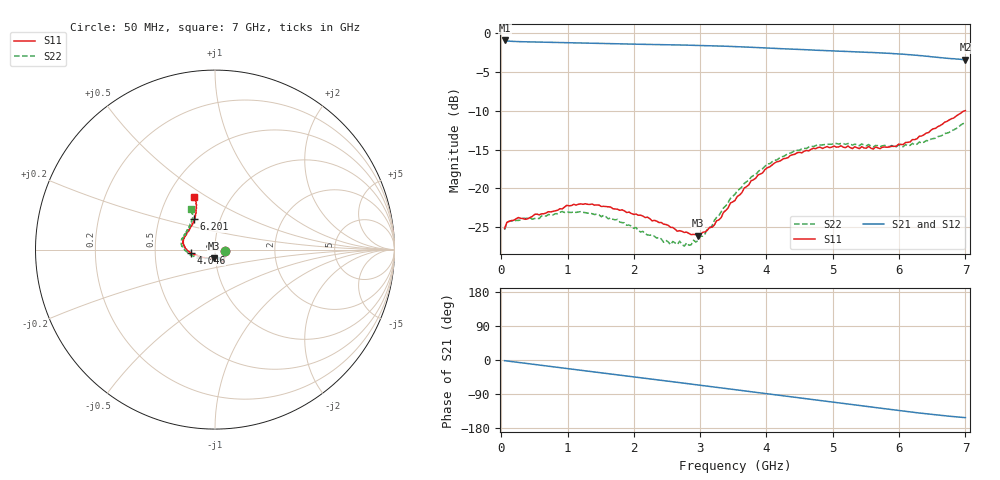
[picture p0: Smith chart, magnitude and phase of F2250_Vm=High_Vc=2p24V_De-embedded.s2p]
! Integrated Device Technology
! Corporate Headquarters
! 6024 Silver Creek Valley Road
! San Jose, CA 95138  USA
! Phone:  1-408-284-8200
! Toll Free:  1-800-223-1366
! Webpage:  http://www.idt.com/
! Timing and RF Division
! 515 Groton Road, Suite 102
! Westford, MA 01886-6024
! Device:  F2250
! Description: Voltage Variable RF Attenuator
! Frequency:  50.0 -  6000.00 MHz
! Package:  3x3 mm Thin QFN Plastic Package: 16 pin
! Ports:  2 RF, 3 DC
!  Pin  1  = GND
!  Pin  2  = NC
!  Pin  3  = RF1  = Port 1
!  Pin  4  = NC
!  Pin  5  = GND
!  Pin  6  = GND
!  Pin  7  = GND
!  Pin  8  = GND
!  Pin  9  = NC
!  Pin 10  = RF2  = Port 2
!  Pin 11  = NC
!  Pin 12  = GND
!  Pin 13  = GND
!  Pin 14  = VCNTRL
!  Pin 15  = VDD
!  Pin 16  = VMODE
! Vcntrl:  2.240 Volts
! Vmode:  +3.300 Volts
! Vdd:  +3.30  Volts
! Current:  1.315 mA
! Data:  The device was measured on a the F2250 evaluation board which has
!  individual transmission lines to the RF pins.  Data was collected
!  using a calibrated network analyzer.  The evaluation board was
!  de-embedded using a TRL calibration technique.
!  The reference plane is the edge of the package pin.
! Misc:  SN 10
!  Action Tracker AT0258
! Date Measured:  2014-11-26
! Date:  2015-10-15  MJV
! Note:
!  Integrated Device Technology supplies this data as a sample of measured
!  data at the package pin for this product.  Your particular data for this
!  product may vary.
!  Data was taken at 25 degrees C.
!  Integrated Device Technology reserves the right to change this data at anytime.
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# GHz S dB R 50
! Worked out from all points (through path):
!   201 points, 50 MHz to 7 GHz, reference 50 ohm
!   highest |S21| = -0.92 dB at 50 MHz (marker M1); lowest = -3.4 dB at 7 GHz (marker M2)
!   group delay of S21, straight-line fit = 61.1 ps
!   lowest |S11| = -26.1 dB at 2.969 GHz (marker M3), VSWR 1.10, Z = 49.3 - j4.87 ohm
!   |S11| at or under -10 dB: start of sweep to 6.992 GHz
!   |S22| runs from -27.5 to -11.5 dB; largest |S21 - S12| = 0.0019
!   S11 on the Smith chart (normalised r, x): 50 MHz: 1.11, -0.02; 4.046 GHz: 0.76, -0.03; 6.201 GHz: 0.75, +0.27; 7 GHz: 0.68, +0.44
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0.05  -25.19 -10.1  -0.92 -1.8  -0.92 -1.8  -25.36 -10.5
0.1195  -24.28 -9.8  -1.02 -3.2  -1.01 -3.2  -24.25 -8.6
0.91875  -22.67 -48.6  -1.20 -21.0  -1.20 -21.1  -23.00 -50.1
1.2315  -22.07 -56.4  -1.27 -27.9  -1.27 -27.9  -23.12 -60.6
1.75275  -22.71 -63.3  -1.36 -39.1  -1.36 -39.1  -24.01 -67.3
2.37825  -24.43 -63.2  -1.45 -52.8  -1.45 -52.8  -26.35 -67.5
2.552  -25.05 -67.9  -1.48 -56.6  -1.48 -56.7  -27.28 -74.0
2.691  -25.47 -75.6  -1.50 -59.8  -1.50 -59.8  -26.84 -81.5
2.7605  -25.71 -77.7  -1.51 -61.3  -1.51 -61.3  -27.48 -85.9
2.969  -26.12 -95.0  -1.55 -66.0  -1.55 -66.0  -26.77 -104.8
3.21225  -24.76 -124.9  -1.61 -71.5  -1.61 -71.5  -24.15 -129.5
3.4555  -21.91 -146.3  -1.69 -76.9  -1.69 -77.0  -21.30 -144.8
3.525  -21.58 -150.6  -1.71 -78.5  -1.71 -78.6  -20.77 -148.1
3.76825  -19.04 -163.2  -1.80 -84.0  -1.80 -84.0  -18.56 -159.2
4.04625  -17.25 -172.8  -1.91 -90.2  -1.91 -90.2  -16.84 -169.6
4.4285  -15.61 177.0  -2.06 -98.6  -2.06 -98.6  -15.12 179.0
4.7065  -14.84 169.9  -2.16 -104.8  -2.16 -104.8  -14.61 173.2
5.054  -14.69 161.8  -2.29 -112.5  -2.28 -112.5  -14.22 166.1
5.85325  -14.67 135.8  -2.59 -130.0  -2.59 -130.1  -14.62 147.4
6.20075  -13.72 124.2  -2.79 -137.7  -2.80 -137.8  -14.21 138.3
6.54825  -12.27 116.0  -3.07 -144.7  -3.07 -144.8  -13.55 127.0
7  -9.98 111.1  -3.39 -152.1  -3.40 -152.2  -11.53 120.7
